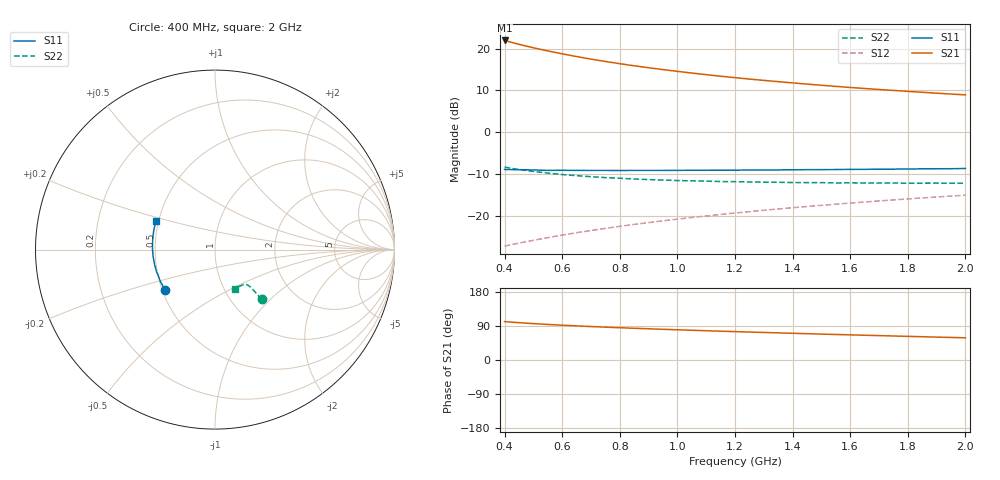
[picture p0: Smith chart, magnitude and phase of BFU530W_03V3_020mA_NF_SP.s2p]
! Filename:  P:\Prog\Test\Noise\ATS_data\Testdata_Net\06 Compressed Noise after Statistics\BFU530W_APM2013_09_A05_03p3V_020mA_NF_CM01_D.sf
! Date/Time: Tue 26/Mar/2013 18:06:06
! BFU530W_APM2013_09_A05_03p3V_1to25mA_NF_CM01_Bias8_R.sf
! Noise Parameter Data File
! BFU530W_APM2013_09_A05_03p3V_1to25mA_NF_CM01
! Date/time: Thu Mar 21 19:18:02 2013
! VAR V_out= 3.300000
! VAR I_out= 20.000000
! VAR V_in= 0.847100
! VAR I_in= 0.221350
! Device data file deembeded for feedlines and parallel
! Original file: \06 Compressed Noise after Statistics\BFU530W_APM2013_09_A05_03p3V_020mA_NF_CM01_R.sf
! Feed-files: PR019V01_070313_Feed1.s2p, PR019V01_070313_Feed2.s2p
! Parallel-file: PR019V01_070313_Par.s2p
# MHz S MA R 50
!  Freq-MHz  S11-mag  S11-arg  S21-mag  S21-arg  S12-mag  S12-arg  S22-mag  S22-arg
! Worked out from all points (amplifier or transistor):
!   37 points, 400 MHz to 2 GHz, reference 50 ohm
!   highest |S21| = 21.9 dB at 400 MHz (marker M1)
!   |S21| within 3 dB of that: start of sweep to 585.3 MHz
!   unconditionally stable (mu >= 1): 967.5 MHz to end of sweep
!   at 500 MHz: K = 0.89, MSG = 23.1 dB, |S12| = -25.9 dB
!   at 1.1 GHz: K = 1.01, MAG = 16.3 dB, |S12| = -20.1 dB
!   at 2 GHz: K = 1.01, MAG = 11.6 dB, |S12| = -15.1 dB
!   lowest NFmin = 0.97 dB at 433 MHz
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400  0.3564 -141.2  12.49 101.3  0.04294 65.5  0.3801 -46.7
420  0.3552 -143.6  11.96 100.1  0.04445 65.8  0.3699 -46.8
440  0.3537 -145.8  11.47 99.0  0.04594 66.2  0.3604 -46.8
460  0.3529 -147.7  11.01 98.0  0.04746 66.5  0.3525 -46.8
500  0.351 -151.5  10.2 96.0  0.05045 67.1  0.3372 -46.7
550  0.3475 -155.4  9.357 93.8  0.05435 67.8  0.3222 -46.6
600  0.3481 -159.0  8.638 91.8  0.05829 68.3  0.3094 -46.5
650  0.347 -162.3  8.011 90.0  0.06218 68.8  0.3001 -46.5
700  0.3467 -165.2  7.469 88.3  0.06615 69.2  0.2917 -46.6
750  0.3466 -167.8  6.997 86.7  0.07015 69.6  0.2844 -46.6
800  0.3459 -170.4  6.58 85.2  0.07419 69.9  0.2795 -46.9
850  0.3467 -172.6  6.213 83.7  0.07823 70.1  0.2736 -47.1
950  0.3468 -176.7  5.593 81.0  0.08643 70.4  0.2662 -47.7
1050  0.3482 179.6  5.085 78.5  0.09467 70.6  0.2603 -48.4
1150  0.3495 176.0  4.661 76.1  0.1029 70.6  0.2553 -49.5
1200  0.3495 174.5  4.479 74.9  0.1071 70.5  0.2544 -50.2
1250  0.3501 172.9  4.306 73.8  0.1113 70.5  0.252 -50.7
1350  0.3516 170.2  4.009 71.6  0.1198 70.3  0.2501 -52.0
1500  0.3543 165.9  3.63 68.3  0.1324 69.8  0.2475 -54.5
1650  0.3572 162.0  3.32 65.4  0.1451 69.2  0.2452 -56.7
1750  0.3593 159.8  3.15 63.4  0.1538 68.8  0.2449 -58.4
2000  0.3659 154.0  2.785 58.5  0.1752 67.4  0.2444 -63.2
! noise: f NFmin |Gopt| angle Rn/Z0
400  1.025  0.2645  -172.6  0.0744
460  1.014  0.2907  -172  0.0681
600  1.028  0.2807  -167.6  0.0741
800  1.055  0.3155  -164.8  0.0681
1000  1.08  0.3225  -161.3  0.0696
1200  1.086  0.3416  -157.2  0.0726
1400  1.128  0.3605  -154  0.0713
1600  1.157  0.3669  -149  0.0775
1800  1.198  0.3704  -143.8  0.0879
2000  1.223  0.3751  -142.2  0.0945
